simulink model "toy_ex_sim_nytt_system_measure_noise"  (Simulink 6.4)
settings: Solver=ode4  StartTime=0.0  StopTime=simtid  FixedStep=.05  RelTol=1e-5
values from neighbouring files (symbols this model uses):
  alpha = -0.9    [bounds.m]    (also in real_ex_linkomb_W_and_DP.m = 1; real_ex_linkomb_W_and_RHOT.m = -0.2; real_ex_without_noise_z_30.m = -6:0.01:4; toy_ex_nytt_system.m)
  den_G1 = [-1 1]    [bounds.m]    (also in toy_ex_nytt_system.m; toy_ex_nytt_system_without_noise.m; toy_ex_nytt_system_with_disturbance.m; toy_ex_nytt_system_with_measure_noise.m)
  den_G2 = [-1 1]    [bounds.m]    (also in toy_ex_nytt_system.m; toy_ex_nytt_system_without_noise.m; toy_ex_nytt_system_with_disturbance.m; toy_ex_nytt_system_with_measure_noise.m)
  K_indre = 10    [real_ex_linkomb_W_and_DP.m]    (also in real_ex_linkomb_W_and_RHOT.m = 5; toy_ex_nytt_system.m = 50; toy_ex_nytt_system_without_noise.m = 20; toy_ex_nytt_system_with_disturbance.m = 50)
  K_ytre = 0.01    [real_ex_linkomb_W_and_DP.m]    (also in real_ex_linkomb_W_and_RHOT.m; toy_ex_nytt_system.m = 0.1; toy_ex_nytt_system_without_noise.m = 0.1; toy_ex_nytt_system_with_disturbance.m = 0.1)
  num_G1 = 5*[-1.5 1]    [bounds.m]    (also in toy_ex_nytt_system.m; toy_ex_nytt_system_without_noise.m; toy_ex_nytt_system_with_disturbance.m; toy_ex_nytt_system_with_measure_noise.m)
  num_G2 = 5*[-0.5 1]    [bounds.m]    (also in toy_ex_nytt_system.m; toy_ex_nytt_system_without_noise.m; toy_ex_nytt_system_with_disturbance.m; toy_ex_nytt_system_with_measure_noise.m)
  Ti = 100    [real_ex_linkomb_W_and_DP.m]    (also in real_ex_linkomb_W_and_RHOT.m = 100000; toy_ex_nytt_system.m = 10; toy_ex_nytt_system_without_noise.m = 10; toy_ex_nytt_system_with_disturbance.m = 10)

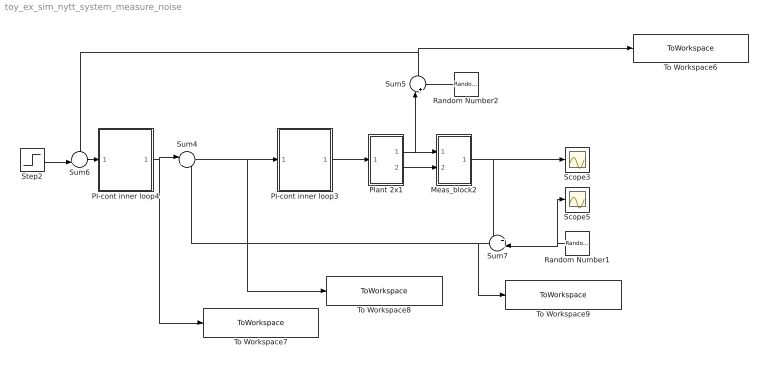
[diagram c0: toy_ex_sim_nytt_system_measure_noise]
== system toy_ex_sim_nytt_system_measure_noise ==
  Meas_block2 : Subsystem
  PI-cont inner loop3 : Subsystem
  PI-cont inner loop4 : Subsystem
  Plant 2x1 : Subsystem
  Random Number1 : RandomNumber  Orientation=left  Variance=(.5* 0.1*0.05)^2  SampleTime=0
  Random Number2 : RandomNumber  Orientation=left  Variance=(.5* 0.05)^2  SampleTime=0
  Scope3 : Scope
  Scope5 : Scope
  Step2 : Step  SampleTime=0
  Sum4 : Sum  Inputs=|+-
  Sum5 : Sum  Orientation=up  Inputs=|++
  Sum6 : Sum  Inputs=-+|
  Sum7 : Sum  Orientation=left  Inputs=++|
  To Workspace6 : ToWorkspace  VariableName=meas_y1  SampleTime=-1  SaveFormat=Structure With Time
  To Workspace7 : ToWorkspace  VariableName=meas_u_outer  SampleTime=-1  SaveFormat=Structure With Time
  To Workspace8 : ToWorkspace  VariableName=meas_u_inner  SampleTime=-1  SaveFormat=Structure With Time
  To Workspace9 : ToWorkspace  VariableName=meas_linkomb  SampleTime=-1  SaveFormat=Structure With Time
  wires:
  Plant 2x1/2(y2) -> Meas_block2/2(In2)
  Plant 2x1/1("y1 ") -> Meas_block2/1(In1), Sum5/1
  Meas_block2/1(Out1) -> Sum7/1, Scope3/1
  Sum4/1 -> To Workspace8/1, PI-cont inner loop3/1(In1)
  PI-cont inner loop3/1(Out1) -> Plant 2x1/1(In1)
  PI-cont inner loop4/1(Out1) -> To Workspace7/1, Sum4/1
  Step2/1 -> Sum6/2
  Sum6/1 -> PI-cont inner loop4/1(In1)
  Sum7/1 -> Sum4/2, To Workspace9/1
  Random Number1/1 -> Scope5/1, Sum7/2
  Random Number2/1 -> Sum5/2
  Sum5/1 -> To Workspace6/1, Sum6/1

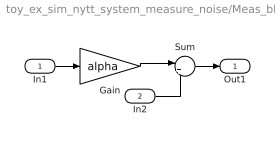
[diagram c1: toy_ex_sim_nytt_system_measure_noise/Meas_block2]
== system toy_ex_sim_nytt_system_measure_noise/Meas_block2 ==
  In1 : Inport
  In2 : Inport  Port=2
  Gain : Gain  Gain=alpha
  Sum : Sum  Inputs=|++
  Out1 : Outport
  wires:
  Gain/1 -> Sum/1
  In1/1 -> Gain/1
  Sum/1 -> Out1/1
  In2/1 -> Sum/2

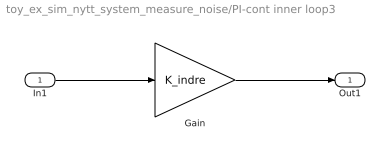
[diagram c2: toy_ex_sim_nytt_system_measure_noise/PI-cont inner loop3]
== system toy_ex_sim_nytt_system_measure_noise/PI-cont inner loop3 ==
  In1 : Inport
  Gain : Gain  Gain=K_indre
  Out1 : Outport
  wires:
  Gain/1 -> Out1/1
  In1/1 -> Gain/1

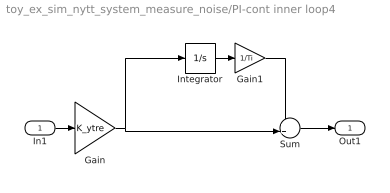
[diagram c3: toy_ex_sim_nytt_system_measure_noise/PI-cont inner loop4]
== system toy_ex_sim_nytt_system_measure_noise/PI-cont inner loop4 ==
  In1 : Inport
  Gain : Gain  Gain=K_ytre
  Gain1 : Gain  Gain=1/Ti
  Integrator : Integrator
  Sum : Sum  Inputs=++|
  Out1 : Outport
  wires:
  Sum/1 -> Out1/1
  Gain1/1 -> Sum/1
  Integrator/1 -> Gain1/1
  In1/1 -> Gain/1
  Gain/1 -> Sum/2, Integrator/1

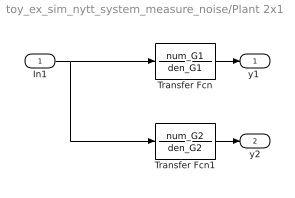
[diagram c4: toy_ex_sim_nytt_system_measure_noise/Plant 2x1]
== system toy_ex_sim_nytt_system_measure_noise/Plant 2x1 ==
  In1 : Inport
  Transfer Fcn : TransferFcn  Numerator=num_G1  Denominator=den_G1
  Transfer Fcn1 : TransferFcn  Numerator=num_G2  Denominator=den_G2
  "y1 " : Outport
  y2 : Outport  Port=2
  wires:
  In1/1 -> Transfer Fcn1/1, Transfer Fcn/1
  Transfer Fcn/1 -> "y1 "/1
  Transfer Fcn1/1 -> y2/1
